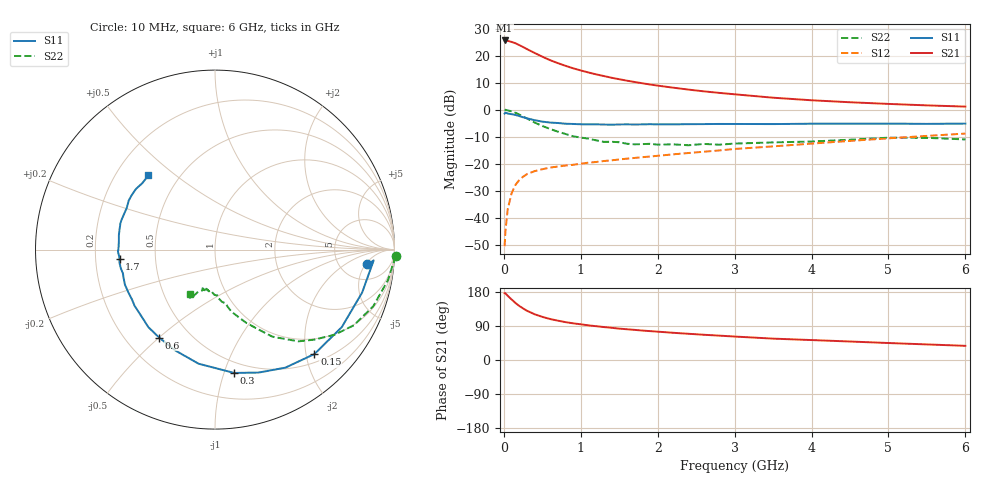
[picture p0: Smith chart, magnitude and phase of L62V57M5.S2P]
!  INFINEON TECHNOLOGIES Small Signal Semiconductors
! BFR380L3 , Si-NPN RF-Transistor in TSLP-3-1
!  Vce=2.5 V,  Ic=7.5 mA
! Common Emitter S-Parameters:  07. March 2005
#  GHz  S  MA  R  50
! f  S11  S21  S12  S22
! GHz  Mag  Ang  Mag  Ang  Mag  Ang  Mag  Ang
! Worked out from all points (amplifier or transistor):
!   36 points, 10 MHz to 6 GHz, reference 50 ohm
!   highest |S21| = 25.6 dB at 10 MHz (marker M1)
!   |S21| within 3 dB of that: start of sweep to 287.9 MHz
!   unconditionally stable (mu >= 1): 2.259 GHz to 4.755 GHz
!   at 250 MHz: K = 0.22, MSG = 24.0 dB, |S12| = -24.8 dB
!   at 1.4 GHz: K = 0.85, MSG = 15.3 dB, |S12| = -18.7 dB
!   at 6 GHz: K = 0.95, MSG = 5.0 dB, |S12| = -8.8 dB
!   S11 on the Smith chart (normalised r, x): 10 MHz: 9, -5; 150 MHz: 0.66, -2.17; 300 MHz: 0.41, -1.08; 600 MHz: 0.34, -0.50; 1.7 GHz: 0.30, -0.05; 6 GHz: 0.34, +0.40
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0.01  0.8505 -5.6  19.16 176.2  0.003 81.4  1.009 -2.1
0.02  0.8861 -3.9  19.11 176.0  0.0055 87.2  0.9967 -4.3
0.05  0.8539 -16.3  18.84 169.5  0.0144 82.9  0.978 -10.1
0.1  0.828 -31.4  18.02 159.9  0.0283 74.5  0.9365 -19.7
0.15  0.8035 -46.4  17.02 150.7  0.0406 67.2  0.881 -28.6
0.2  0.7657 -59.2  15.75 142.7  0.05 62.9  0.8173 -35.5
0.25  0.7271 -70.4  14.5 136.1  0.0578 57.4  0.7468 -42.2
0.3  0.6954 -81.2  13.28 130.0  0.0644 54.2  0.6912 -47.7
0.4  0.6423 -98.2  11.24 120.7  0.0733 49.3  0.5813 -56.6
0.5  0.6041 -111.4  9.602 113.9  0.0795 46.5  0.5018 -61.8
0.6  0.5808 -122.4  8.294 108.2  0.0852 45.2  0.4425 -67.0
0.7  0.5696 -130.7  7.31 103.9  0.089 44.9  0.3948 -71.1
0.8  0.5525 -138.3  6.516 100.0  0.0929 44.5  0.3572 -75.2
1.1  0.5384 -154.3  4.897 91.4  0.1051 46.3  0.2929 -82.6
1.4  0.5299 -165.4  3.914 85.0  0.1161 48.4  0.256 -88.2
1.7  0.5339 -174.3  3.265 79.5  0.1286 50.7  0.2297 -94.8
2.2  0.5376 175.0  2.565 71.8  0.1498 54.0  0.2292 -100.0
2.8  0.547 164.5  2.053 64.3  0.177 57.3  0.226 -107.8
3.5  0.5438 154.7  1.673 56.4  0.2104 58.4  0.2491 -111.0
4.5  0.5545 147.0  1.378 48.8  0.2657 60.3  0.2794 -114.4
5.5  0.5486 137.7  1.206 41.1  0.3286 59.0  0.3026 -117.5
6  0.5556 132.0  1.145 37.4  0.3629 57.7  0.2827 -119.7
